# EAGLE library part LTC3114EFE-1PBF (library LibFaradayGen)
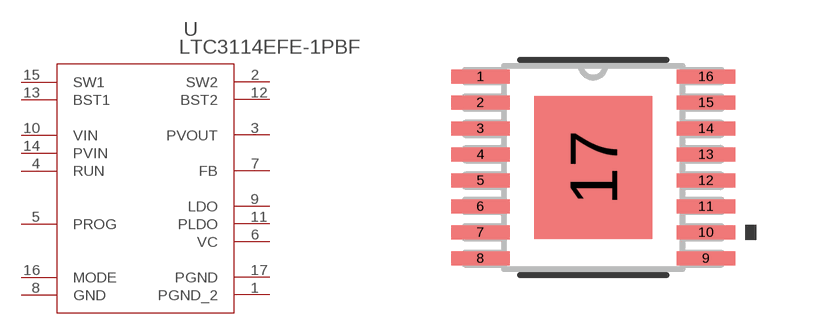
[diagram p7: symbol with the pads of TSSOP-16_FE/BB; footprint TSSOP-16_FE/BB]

Designator prefix U

## LTC3114EFE-1PBF (MANUFACTURER_PART_NUMBER: LTC3114EFE1#PBF; VENDOR: Linear Technology)  [TSSOP-16_FE/BB]
1  PGND_2  pwr
2  SW2  pas
3  PVOUT  out
4  RUN  in
5  PROG  out
6  VC  out
7  FB  in
8  GND  pwr
9  LDO  in
10  VIN  in
11  PLDO  out
12  BST2  pas
13  BST1  pas
14  PVIN  in
15  SW1  pas
16  MODE  pas
17  PGND  pwr

## Footprint TSSOP-16_FE/BB (pad centres in mm)
smd 1.473 x 0.356: 1 -2.819,2.276; 2 -2.819,1.626; 3 -2.819,0.975; 4 -2.819,0.325; 5 -2.819,-0.325; 6 -2.819,-0.975; 7 -2.819,-1.626; 8 -2.819,-2.276; 9 2.819,-2.276; 10 2.819,-1.626; 11 2.819,-0.975; 12 2.819,-0.325; 13 2.819,0.325; 14 2.819,0.975; 15 2.819,1.626; 16 2.819,2.276
smd 2.946 x 3.581: 17 0,0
